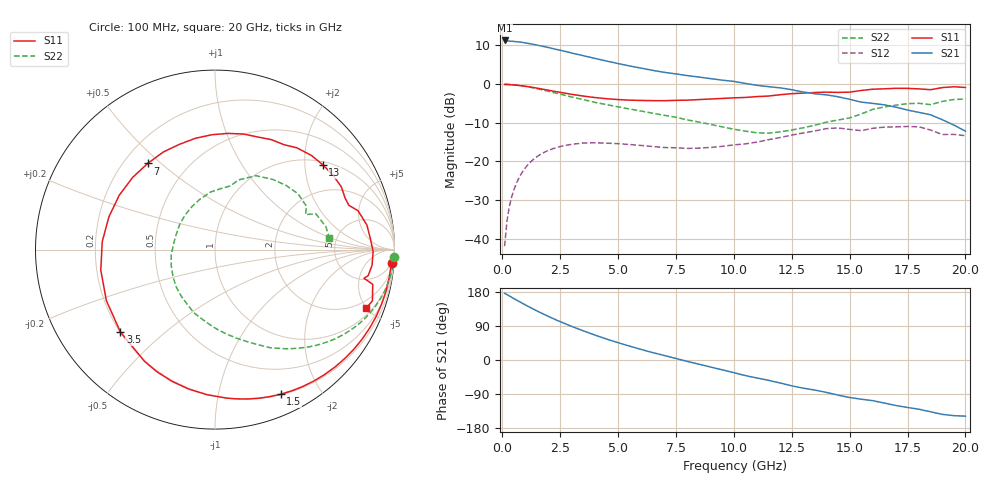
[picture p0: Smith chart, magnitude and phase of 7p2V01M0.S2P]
! Infineon Technologies  Discrete & RF Semiconductors
! bfp620
! VCE =  2.0 V,  IC =  1.0 mA
! Common Emitter S-Parameters:  Sep 2002
# GHz  S  MA  R  50
!  f  S11  S21  S12  S22
! GHz  MAG  ANG  MAG  ANG  MAG  ANG  MAG  ANG
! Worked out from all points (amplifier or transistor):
!   59 points, 100 MHz to 20 GHz, reference 50 ohm
!   highest |S21| = 11.3 dB at 100 MHz (marker M1)
!   |S21| within 3 dB of that: start of sweep to 2.842 GHz
!   unconditionally stable (mu >= 1): 6.311 GHz to 15.75 GHz; 17.89 GHz to 18.99 GHz; 19.56 GHz to end of sweep
!   at 1 GHz: K = 0.10, MSG = 16.1 dB, |S12| = -21.6 dB
!   at 5.5 GHz: K = 0.83, MSG = 10.2 dB, |S12| = -15.6 dB
!   at 20 GHz: K = 1.33, MAG = -2.9 dB, |S12| = -13.3 dB
!   S11 on the Smith chart (normalised r, x): 100 MHz: 5, -26; 1.5 GHz: 0.21, -1.54; 3.5 GHz: 0.20, -0.36; 7 GHz: 0.30, +0.45; 13 GHz: 1.09, +2.47; 20 GHz: 1.39, -4.97
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0.1  0.9863 -4.2  3.663 176.1  0.008 81.9  0.9992 -2.4
0.2  0.9833 -9.0  3.621 172.7  0.0168 84.0  0.9961 -4.8
0.3  0.9804 -13.6  3.595 169.2  0.0256 82.4  0.9918 -7.1
0.5  0.972 -22.6  3.557 162.2  0.0428 77.0  0.9797 -11.6
1  0.935 -44.5  3.406 145.3  0.0828 62.4  0.9327 -22.3
1.5  0.8851 -65.5  3.19 129.5  0.1152 48.9  0.8701 -31.8
1.9  0.8411 -81.5  3.007 117.7  0.1349 39.3  0.8171 -38.6
2.4  0.7906 -100.7  2.777 103.8  0.1527 28.7  0.7526 -46.1
3  0.7362 -122.2  2.516 88.6  0.1661 17.4  0.6804 -54.3
3.5  0.6987 -139.0  2.327 76.9  0.1728 9.1  0.629 -60.5
4  0.6687 -154.8  2.146 65.8  0.1739 1.5  0.5798 -65.9
5  0.6298 176.0  1.842 45.7  0.1694 -9.6  0.5075 -76.4
6  0.6135 150.4  1.606 27.8  0.1605 -17.5  0.4473 -87.8
7  0.6092 128.0  1.417 11.8  0.1511 -21.5  0.3942 -100.4
9  0.6405 91.4  1.174 -18.7  0.1515 -23.1  0.3009 -135.5
10.5  0.6712 69.2  1.019 -41.2  0.1685 -25.8  0.2461 -172.7
13  0.7641 38.2  0.789 -74.4  0.233 -37.7  0.2719 118.2
13.5  0.7771 32.3  0.748 -79.4  0.2474 -42.4  0.2934 106.4
16  0.8574 9.2  0.562 -107.3  0.2679 -66.4  0.4706 61.1
17  0.8812 -0.7  0.502 -120.1  0.2792 -78.8  0.5335 42.1
18.5  0.8453 -10.9  0.4 -136.7  0.2539 -102.1  0.5413 21.1
20  0.9036 -21.2  0.246 -148.2  0.2151 -108.2  0.6403 5.8
